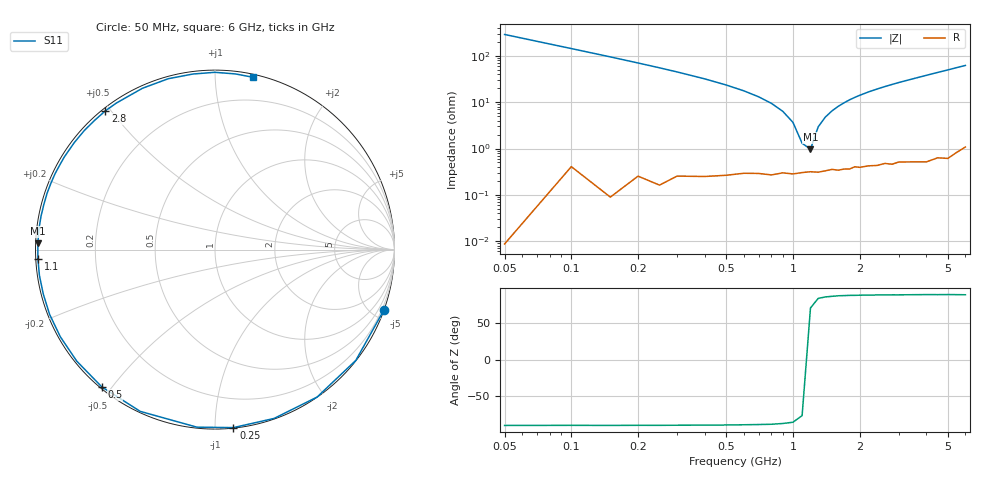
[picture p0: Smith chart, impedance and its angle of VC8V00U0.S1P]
! Infineon Technologies  Discrete & RF Semiconductors
! BBY 56-03
! Si Tuning Diode in SOD323
! VR = 8 V
! S-Parameters:  June  1999
# GHz  S  MA  R  50
!  f  S11
! GHz  MAG  ANG
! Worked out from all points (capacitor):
!   34 points, 50 MHz to 6 GHz, reference 50 ohm
!   read as one part to ground: C = 10.9 pF near 50 MHz
!   lowest |Z| = 969 mohm at 1.2 GHz (marker M1)
!   series resonance near 1.158 GHz, so ESL is about 1.7 nH
!   S11 on the Smith chart (normalised r, x): 50 MHz: 0.00, -5.82; 250 MHz: 0.00, -1.11; 500 MHz: 0.01, -0.47; 1.1 GHz: 0.01, -0.03; 2.8 GHz: 0.01, +0.48; 6 GHz: 0.02, +1.25
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0.05  1 -19.5
0.1  0.9983 -38.2
0.15  0.9992 -55.3
0.2  0.9966 -70.7
0.25  0.9971 -84.1
0.3  0.9944 -95.8
0.4  0.9929 -114.8
0.5  0.9914 -129.5
0.6  0.9896 -141.1
0.7  0.9892 -150.6
0.8  0.9897 -158.6
0.9  0.9883 -165.5
1.1  0.9879 -177.1
1.2  0.9875 177.9
1.4  0.987 169.1
1.6  0.9868 161.5
1.8  0.9863 154.6
2  0.9855 148.5
2.2  0.9849 142.8
2.4  0.9851 137.7
2.8  0.9852 128.3
3  0.9842 123.9
3.5  0.9856 114.2
4  0.987 105.3
4.5  0.9859 97.2
5  0.9878 90.1
5.5  0.9853 83.3
6  0.9832 77.4
